FUNCTION_BLOCK Siemens_AWL2_src
TITLE = Ampelschaltung einfach
// taken from the Siemens S7 Help/Instruction List examples
// Steuerung einer Ampelanlage fuer einen Fussgaengeruebergang
// an der Hauptstrasse

{S7_pdiag := 'true'} //Systemattribut fuer Bausteine
AUTHOR : SIEMENS
FAMILY : Ampel
NAME : Siemens_AWL2_src
VERSION : 1.3

VAR_INPUT

starter : BOOL := FALSE; // Ueberquerungswunsch Fußgaenger
t_dur_y_car : TIMER; // Zeitdauer Gruen Fussgaenger
t_next_r_car : TIMER; // Zeitdauer zwischen Rot fuer Auto
t_dur_r_car : TIMER;
anz {S7_server := 'alarm_archiv'; S7_a_type := 'alarm_8'} :DWORD;
// Anzahl Autos
// anz besitzt Systemattribute fuer Parameter

END_VAR
VAR_OUTPUT

g_car : BOOL := FALSE; // GRUEN fuer Autos

END_VAR
VAR
condition : BOOL := FALSE; // Vormerkung Rot fuer Autos
END_VAR

BEGIN
NETWORK
TITLE = Vormerkung Rot fuer Strassenverkehr
// Nach Einhalten eines Mindestzeitabstands wird durch
//den Signalwunsch am Fussgaengeruebergang die
//Vormerkung Rot fuer den Strassenverkehr gebildet.
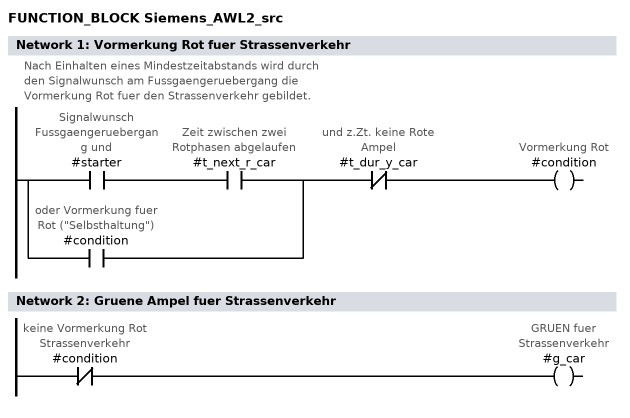
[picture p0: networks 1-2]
U(;
U #starter; // Signalwunsch Fussgaengeruebergang und
U #t_next_r_car; // Zeit zwischen zwei Rotphasen abgelaufen
O #condition; // oder Vormerkung fuer Rot ("Selbsthaltung")
);
UN #t_dur_y_car; // und z.Zt. keine Rote Ampel
= #condition; // Vormerkung Rot
NETWORK
TITLE = Gruene Ampel fuer Strassenverkehr
UN #condition; // keine Vormerkung Rot Strassenverkehr
= #g_car; // GRUEN fuer Strassenverkehr
NETWORK
TITLE = Dauer fuer Gelbphase Autos
// weiteres Programm zur Realisierung
// der Ampelschaltung

END_FUNCTION_BLOCK

FUNCTION_BLOCK FB 10
VAR_INPUT
para1 : bool;
para2: bool;
end_var
begin
end_function_block

data_block db 10
fb10
begin
end_data_block

data_block db 6
fb6
begin
end_data_block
